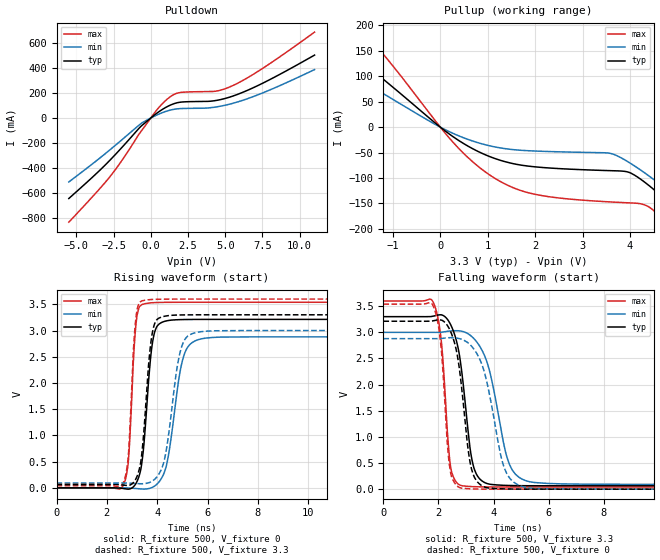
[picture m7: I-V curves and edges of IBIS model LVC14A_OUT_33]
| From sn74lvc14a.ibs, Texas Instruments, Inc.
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[Model]   LVC14A_OUT_33
Model_type  Output
Vref =   0
Rref =   500
Cref =   50p
Vmeas =   1.5
| variable   typ   min   max
C_comp   7.71pF   3.93pF   12.74pF
| C_pullup   6.91pF   3.93pF   8.21pF
| C_pulldown   8.52pF   4.17pF   12.74pF
[Temperature Range]   40   100   -40
| Ambient temperature   25   85   -40
[Voltage range]   3.3   3   3.6
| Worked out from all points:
|   slope of the pulldown table from 0 to 0.495 V, typ, clamps not added: 10.7 ohm
|   slope of the pullup table from 0 to 0.495 V, typ, clamps not added: 15.2 ohm
|   rising waveform, R_fixture 500, V_fixture 0: 20-80 % time 326ps typ, 514ps min, 224ps max; typ from 0 V to 3.21 V
|   falling waveform, R_fixture 500, V_fixture 3.3: 20-80 % time 436ps typ, 686ps min, 284ps max; typ from 3.3 V to 0.065 V
|   rising waveform, R_fixture 500, V_fixture 3.3: 20-80 % time 317ps typ, 492ps min, 219ps max; typ from 0.065 V to 3.3 V
|   falling waveform, R_fixture 500, V_fixture 0: 20-80 % time 428ps typ, 665ps min, 278ps max; typ from 3.21 V to 0 V
[Pulldown]
| LVC14A_OUT_33
|   Voltage   I(typ)   I(min)   I(max)
-5.5V     -645.8mA   -513mA     -835.8mA
-3.645V   -444.9mA   -342.7mA   -596.4mA
-2.71V    -334.7mA   -252.1mA   -466mA
-1.89V    -230mA     -169.6mA   -332.4mA
-620mV    -62.41mA   -41.52mA   -102.1mA
455mV     42.83mA    26.93mA    71.74mA
1.215V    98.07mA    60.46mA    162.3mA
1.91V     125.9mA    75.23mA    203.5mA
4.31V     139.6mA    87.57mA    214.6mA
5.45V     173.8mA    116.3mA    257.3mA
7.53V     280.4mA    202.4mA    399.9mA
11V       505.3mA    389mA      689.8mA
[Pullup]
| LVC14A_OUT_33
|   Voltage   I(typ)   I(min)   I(max)
-5.5V     404.4mA    310.8mA    569.2mA
-3.515V   265mA      197.3mA    383.4mA
-2.48V    190.1mA    138.3mA    280.1mA
-1.635V   127.1mA    90.28mA    191.1mA
505mV     -33.05mA   -21.44mA   -52.79mA
1.855V    -76.61mA   -46.34mA   -128.9mA
3.7V      -85.85mA   -55.17mA   -147.6mA
4.24V     -103.4mA   -85.4mA    -151mA
4.89V     -155mA     -131.2mA   -201.1mA
5.36V     -197.9mA   -167.7mA   -253.2mA
5.82V     -242.5mA   -205.2mA   -308.1mA
11V       -792.2mA   -667mA     -979.2mA
[Ramp]
| LVC14A_OUT_33
| variable   typ   min   max
dV/dt_r   1.94/3.36E-10   1.74/5.23E-10   2.14/2.39E-10
dV/dt_f   1.96/4.52E-10   1.76/7.00E-10   2.16/2.97E-10
R_load = 500
[Rising Waveform]
| LVC14A_OUT_33
R_fixture =   500
C_fixture =   0
L_fixture =   0
V_fixture =   0
V_fixture_min = 0
V_fixture_max = 0
|   Time   V(typ)   V(min)   V(max)
0s        184.9pV    3.596nV    20.95pV
2.65ns    -12.61mV   490.2uV    46.54mV
2.855ns   -24.76mV   -2.485mV   522mV
3.185ns   110.2mV    -13.76mV   3.238V
3.615ns   1.755V     -17.77mV   3.52V
4.01ns    3.092V     80.45mV    3.534V
4.395ns   3.187V     490.5mV    3.538V
5.065ns   3.209V     2.531V     3.539V
5.93ns    3.212V     2.856V     3.539V
50ns      3.212V     2.88V      3.539V
[Falling Waveform]
| LVC14A_OUT_33
R_fixture =   500
C_fixture =   0
L_fixture =   0
V_fixture =   3.3
V_fixture_min = 3
V_fixture_max = 3.6
|   Time   V(typ)   V(min)   V(max)
0s        3.3V       3V         3.6V
1.83ns    3.312V     2.999V     3.554V
2.11ns    3.334V     3.003V     2.8V
2.445ns   3.144V     3.027V     415.9mV
2.89ns    2.051V     3.015V     62.39mV
3.17ns    703mV      2.937V     50.59mV
3.42ns    249.4mV    2.795V     45.62mV
4.575ns   70.39mV    479.7mV    42.02mV
5.48ns    65.39mV    127.8mV    41.94mV
50ns      64.52mV    92.1mV     41.93mV
[Rising Waveform]
| LVC14A_OUT_33
R_fixture =   500
C_fixture =   0
L_fixture =   0
V_fixture =   3.3
V_fixture_min = 3
V_fixture_max = 3.6
|   Time   V(typ)   V(min)   V(max)
0s        64.52mV    92.1mV     41.93mV
2.645ns   53.39mV    92.44mV    92.74mV
2.845ns   45.13mV    89.78mV    566.2mV
3.16ns    178.3mV    81.79mV    3.263V
3.515ns   1.37V      82.13mV    3.578V
3.925ns   3.16V      176mV      3.595V
4.32ns    3.275V     614.3mV    3.598V
4.965ns   3.297V     2.682V     3.6V
5.725ns   3.3V       2.977V     3.6V
50ns      3.3V       3V         3.6V
[Falling Waveform]
| LVC14A_OUT_33
R_fixture =   500
C_fixture =   0
L_fixture =   0
V_fixture =   0
V_fixture_min = 0
V_fixture_max = 0
|   Time   V(typ)   V(min)   V(max)
0s        3.212V     2.88V      3.539V
1.82ns    3.222V     2.879V     3.491V
2.085ns   3.236V     2.882V     2.763V
2.425ns   3.034V     2.898V     364.2mV
2.875ns   1.781V     2.861V     16.58mV
3.135ns   555.1mV    2.771V     7.652mV
3.385ns   158mV      2.602V     3.245mV
4.41ns    5.135mV    382.6mV    102.2uV
5.31ns    704.9uV    21.88mV    6.607uV
50ns      1.46nV     8.142nV    72.62pV
